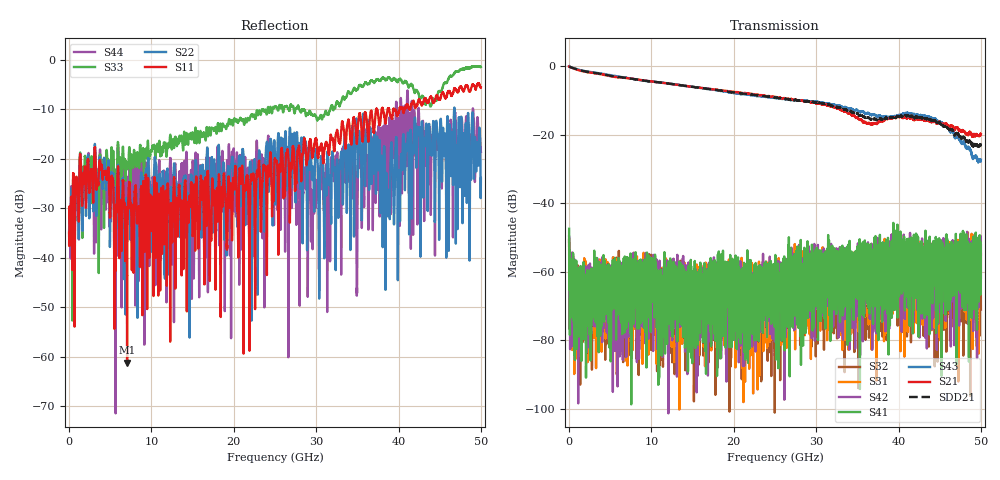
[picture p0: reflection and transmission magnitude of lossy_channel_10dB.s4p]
!Keysight Technologies,N5245A,MY49151038,A.10.65.06
!Date: Wednesday, June 07, 2023 10:56:02
!Correction: S11(Full 4 Port(1,2,3,4))
!S12(Full 4 Port(1,2,3,4))
!S13(Full 4 Port(1,2,3,4))
!S14(Full 4 Port(1,2,3,4))
!S21(Full 4 Port(1,2,3,4))
!S22(Full 4 Port(1,2,3,4))
!S23(Full 4 Port(1,2,3,4))
!S24(Full 4 Port(1,2,3,4))
!S31(Full 4 Port(1,2,3,4))
!S32(Full 4 Port(1,2,3,4))
!S33(Full 4 Port(1,2,3,4))
!S34(Full 4 Port(1,2,3,4))
!S41(Full 4 Port(1,2,3,4))
!S42(Full 4 Port(1,2,3,4))
!S43(Full 4 Port(1,2,3,4))
!S44(Full 4 Port(1,2,3,4))
!S4P File: Measurements: <S11,S12,S13,S14>,
!<S21,S22,S23,S24>,
!<S31,S32,S33,S34>,
!<S41,S42,S43,S44>:
! Created with skrf 1.10.0 (http://scikit-rf.org).
# Hz S RI R 50.0
!freq ReS11 ImS11 ReS12 ImS12 ReS13 ImS13
! ReS14 ImS14
! ReS21 ImS21 ReS22 ImS22 ReS23 ImS23
! ReS24 ImS24
! ReS31 ImS31 ReS32 ImS32 ReS33 ImS33
! ReS34 ImS34
! ReS41 ImS41 ReS42 ImS42 ReS43 ImS43
! ReS44 ImS44
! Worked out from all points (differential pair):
!   5000 points, 10 MHz to 50 GHz, reference 50 ohm
!   strongest paths, dB at 10 MHz, 12.51 GHz, 25.01 GHz, 37.51 GHz, 50 GHz:
!     S21: -0.1, -5.2, -9.0, -16.4, -19.9
!     S43: 0.0, -5.2, -9.3, -14.7, -27.3
!     S41: -47.5, -67.6, -58.9, -55.5, -61.8
!     S42: -49.7, -76.2, -66.1, -56.4, -52.3
!     S31: -50.4, -60.9, -61.9, -61.0, -54.7
!     S32: -50.7, -70.9, -65.6, -67.5, -71.0
!   taken as a pair (ports 1,3 in; 2,4 out), SDD21 dB: -0.1, -5.2, -9.2, -15.6, -22.9
!   lowest |S11| = -61.2 dB at 7.05 GHz (marker M1), VSWR 1.00, Z = 50 - j0.0812 ohm
!   |S11| at or under -10 dB: start of sweep to 37.29 GHz; 38.12 GHz to 38.68 GHz (565 MHz wide, 1.47 % of centre); 39.46 GHz to 40.11 GHz (645.5 MHz wide, 1.62 % of centre)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
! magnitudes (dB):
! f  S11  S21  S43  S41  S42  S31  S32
! 10 MHz  -35.0  -0.1  0.0  -47.5  -49.7  -50.4  -50.7
! 670 MHz  -53.9  -0.8  -0.7  -61.3  -58.2  -61.0  -61.1
! 3.87 GHz  -21.8  -2.4  -2.2  -58.0  -61.0  -61.7  -75.8
! 7.05 GHz  -61.2  -3.5  -3.5  -64.9  -64.9  -58.1  -77.4
! 26.96 GHz  -21.0  -9.6  -9.9  -57.1  -64.6  -62.1  -56.8
! 38.64 GHz  -10.4  -15.4  -15.1  -60.5  -58.1  -59.7  -62.6
! 50 GHz  -5.5  -19.9  -27.3  -61.8  -52.3  -54.7  -71.0
